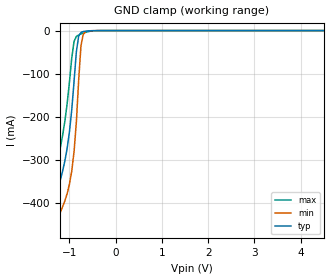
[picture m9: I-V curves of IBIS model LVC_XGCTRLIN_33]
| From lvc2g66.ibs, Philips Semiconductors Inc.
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|   Model LVC_XGCTRLIN_33
[Model]   LVC_XGCTRLIN_33
Model_type   Input
Vinl =   0.8V
Vinh =   2.0V
C_comp   2.96pF   2.12pF   3.91pF
[Model Spec]
| Note: The input and output voltage ratings may be exceeded if the input and
|   output current ratings are observed (please refer to the data sheet)
|   Subparameter   typ   min   max
| Thresholds
Vinh   2.0   2.0   2.0
Vinl   0.8   0.8   0.8
| Overshoot
S_overshoot_high   6.5   6.5   6.5   | Static overshoot
S_overshoot_low   -0.5   -0.5   -0.5
D_overshoot_high   7.2   7.2   7.2   | Dynamic overshoot
D_overshoot_low   -0.95   -0.9   -1.0
D_overshoot_time   3n   3n   3n
|Ambient temperature:   25   85   -40
[Temperature Range]   50   105   -10
[Voltage Range]   3.3V   3.0V   3.6V
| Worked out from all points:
|   GND clamp passes 1 mA (typ) near -0.61 V on its own axis
|Process Range   nominal   slow   fast
[GND_clamp]
| voltage   I(typ)   I(min)   I(max)
-5.5V     -4.562A    -4.619A    -4.506A
-1.45V    -549.4mA   -615.4mA   -482.8mA
-1.4V     -502.2mA   -568.5mA   -435.4mA
-1.35V    -455.9mA   -522.5mA   -388.7mA
-1.3V     -411.6mA   -478.9mA   -343.8mA
-1.1V     -304.2mA   -396.4mA   -212.1mA
-950mV    -185.2mA   -327mA     -64.69mA
-850mV    -49.8mA    -213.4mA   -13.79mA
-750mV    -4.324mA   -35.6mA    -7.884mA
-700mV    -2.27mA    -8.526mA   -5.841mA
-550mV    -593.6uA   -425.2uA   -1.597mA
5.5V      375.8pA    2.471nA    52.76pA
